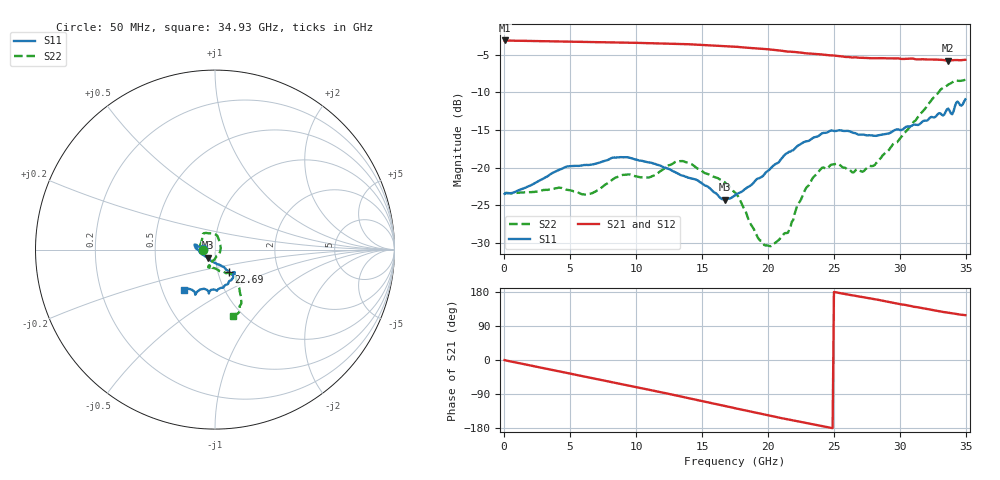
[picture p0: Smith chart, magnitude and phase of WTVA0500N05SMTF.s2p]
! 50 ohm 2-Port S-parameters measured by Modelithics Inc support@modelithics.com  Tampa, FL USA 813-866-6335 (February 2024)
! Smiths Interconnect,  5dB P/N: WTVA0500N05SMTF, Temperature: 125 C
! Board: 10 mil Rogers 4350B, Mounting Pad Dimensions: Length: 15 mils, Width: 25 mils, Gap: 40 mils.
# Hz S RI R 50
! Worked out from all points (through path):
!   352 points, 50 MHz to 34.93 GHz, reference 50 ohm
!   highest |S21| = -3.12 dB at 100 MHz (marker M1); lowest = -5.8 dB at 33.63 GHz (marker M2)
!   group delay of S21, straight-line fit = 19.6 ps
!   lowest |S11| = -24.2 dB at 16.72 GHz (marker M3), VSWR 1.13, Z = 45.8 - j4.15 ohm
!   |S11| at or under -10 dB: start of sweep to end of sweep
!   |S22| runs from -30.4 to -8.3 dB; largest |S21 - S12| = 0.007
!   S11 on the Smith chart (normalised r, x): 50 MHz: 0.87, +0.00; 22.69 GHz: 1.13, -0.29; 34.93 GHz: 0.64, -0.32
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5e7  -0.0671 0.00127  0.6982 -0.0043  0.6974 -0.00438  -0.0668 -0.000639
1e8  -0.0677 0.00098  0.6982 -0.00949  0.6976 -0.00947  -0.0679 -2.1e-05
4.18e9  -0.0953 0.0166  0.5964 -0.342  0.5954 -0.3419  -0.0735 -0.00748
5.8715e9  -0.1006 0.0244  0.5095 -0.4565  0.5088 -0.4562  -0.0665 -0.0075
8.8565e9  -0.1143 0.0277  0.3061 -0.6028  0.3041 -0.6026  -0.0887 0.00767
1.1742e10  -0.1038 0.00465  0.0694 -0.6635  0.0678 -0.6627  -0.0718 0.0599
1.3533e10  -0.0883 -0.00765  -0.0848 -0.6554  -0.0863 -0.6543  -0.0619 0.0918
1.6717e10  -0.0416 -0.0451  -0.3323 -0.5468  -0.3329 -0.5454  0.0109 0.0793
1.7513e10  -0.0236 -0.0615  -0.3846 -0.5049  -0.3846 -0.5036  0.0179 0.0658
1.92045e10  0.0168 -0.0831  -0.473 -0.3974  -0.4721 -0.3971  0.0308 0.0155
2.01995e10  0.0376 -0.0921  -0.5124 -0.3272  -0.5117 -0.3265  0.0282 -0.0108
2.1493e10  0.0604 -0.1103  -0.5403 -0.2344  -0.5398 -0.2327  0.00677 -0.0364
2.2687e10  0.0771 -0.1261  -0.557 -0.1483  -0.5563 -0.1474  -0.0165 -0.0659
2.33835e10  0.0854 -0.1325  -0.5611 -0.1018  -0.5603 -0.1017  -0.0271 -0.0814
2.51745e10  0.1018 -0.143  -0.5521 0.0189  -0.5511 0.0196  -0.0363 -0.1001
2.71645e10  0.109 -0.125  -0.5194 0.1301  -0.5179 0.1321  -0.0221 -0.0915
2.91545e10  0.1008 -0.1355  -0.4748 0.24  -0.4714 0.2441  0.0481 -0.1227
3.1841e10  0.0706 -0.1923  -0.375 0.3648  -0.3723 0.3659  0.1311 -0.2062
3.3632e10  -0.0337 -0.2444  -0.2929 0.4212  -0.2887 0.4232  0.1393 -0.3277
3.39305e10  -0.0609 -0.218  -0.2848 0.431  -0.2808 0.4325  0.1376 -0.3414
3.4229e10  -0.1078 -0.247  -0.2733 0.4402  -0.2689 0.4416  0.1215 -0.3595
3.49255e10  -0.1726 -0.2256  -0.2468 0.4575  -0.2456 0.4567  0.0986 -0.371
